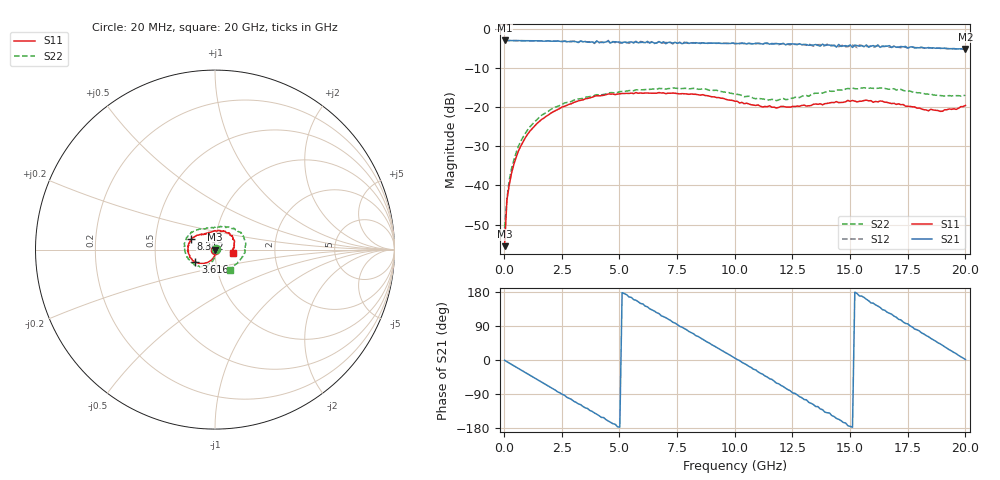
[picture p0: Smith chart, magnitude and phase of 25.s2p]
!Agilent Technologies,N5230A,US43500223,A.07.50.48
!Agilent N5230A: A.07.50.48
!Date: Saturday, September 19, 2015 12:48:16
!Correction: S11(Full 2 Port(1,2))
!S21(Full 2 Port(1,2))
!S12(Full 2 Port(1,2))
!S22(Full 2 Port(1,2))
!S2P File: Measurements: S11, S21, S12, S22:
# Hz S  dB  R 50
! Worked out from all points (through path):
!   201 points, 20 MHz to 20 GHz, reference 50 ohm
!   highest |S21| = -3.03 dB at 20 MHz (marker M1); lowest = -5.2 dB at 20 GHz (marker M2)
!   group delay of S21, straight-line fit = 99.4 ps
!   lowest |S11| = -55.5 dB at 20 MHz (marker M3), VSWR 1.00, Z = 50.2 - j0.055 ohm
!   |S11| at or under -10 dB: start of sweep to end of sweep
!   |S22| runs from -50.8 to -15.1 dB; largest |S21 - S12| = 0.055
!   S11 on the Smith chart (normalised r, x): 20 MHz: 1.00, -0.00; 3.616 GHz: 0.80, -0.11; 8.312 GHz: 0.76, +0.09; 20 GHz: 1.23, -0.05
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2e7  -55.48 -19.0  -3.03 -0.7  -3.03 -0.9  -50.82 11.8
1.199e8  -43.71 -47.9  -3.04 -4.5  -3.04 -4.5  -43.58 -51.6
2.198e8  -39.94 -65.5  -3.05 -8.1  -3.05 -8.1  -38.66 -64.3
7.193e8  -29.97 -92.1  -3.08 -26.1  -3.08 -26.2  -28.76 -88.8
2.3177e9  -20.65 -126.6  -3.16 -84.0  -3.17 -84.2  -19.83 -117.5
3.4166e9  -18.19 -144.2  -3.38 -122.6  -3.38 -123.9  -17.80 -134.5
3.6164e9  -17.82 -148.1  -3.47 -127.9  -3.42 -128.3  -17.43 -137.8
4.9151e9  -16.71 -168.3  -3.43 -176.2  -3.11 -177.0  -16.30 -158.5
6.7133e9  -16.31 173.6  -3.32 122.5  -3.32 122.2  -15.27 176.2
8.3117e9  -16.77 156.4  -3.60 64.3  -3.73 63.6  -15.27 157.5
1.001e10  -18.53 135.6  -3.82 4.6  -3.84 3.9  -16.74 130.7
1.09091e10  -19.60 126.0  -3.73 -26.1  -3.89 -27.4  -17.90 113.0
1.18082e10  -20.24 113.3  -3.82 -61.1  -3.81 -61.1  -18.38 95.0
1.25075e10  -19.85 99.6  -3.89 -86.8  -3.81 -85.9  -17.78 77.6
1.34066e10  -19.31 80.9  -4.21 -117.4  -4.50 -118.9  -16.60 58.6
1.45055e10  -18.88 58.4  -4.04 -156.4  -4.62 -156.2  -15.65 41.0
1.51049e10  -18.33 47.5  -4.80 -177.5  -4.22 178.9  -15.18 32.9
1.57043e10  -18.25 38.9  -4.17 160.4  -4.54 161.7  -15.14 23.1
1.67033e10  -18.99 19.0  -4.35 123.5  -4.78 122.2  -15.48 4.9
1.8002e10  -20.27 -5.1  -4.91 76.7  -4.75 74.7  -16.37 -22.0
1.91009e10  -20.72 -5.9  -5.01 34.9  -5.04 35.0  -17.19 -40.7
2e10  -19.61 -10.7  -5.22 1.5  -5.27 0.6  -17.07 -53.7
